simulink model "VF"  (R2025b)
settings: Solver=FixedStepAuto  StartTime=0.0  StopTime=10.0  FixedStep=1e-4  RelTol=1e-3
undefined symbols (not defined in the file): DiscIntNeverNeededParam, Udc
libraries: fl_lib x6, nesl_utility x6, ee_lib x1

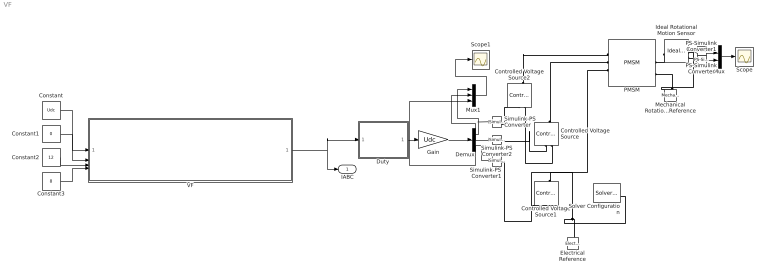
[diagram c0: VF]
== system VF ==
  Constant : Constant  Value=Udc
  Constant1 : Constant  Value=0
  Constant2 : Constant  Value=12
  Constant3 : Constant  Value=8
  Controlled Voltage Source : fl_lib/Electrical/Electrical Sources/Controlled Voltage Source
  Controlled Voltage Source1 : fl_lib/Electrical/Electrical Sources/Controlled Voltage Source
  Controlled Voltage Source2 : fl_lib/Electrical/Electrical Sources/Controlled Voltage Source
  Demux : Demux  Outputs=3
  Duty : Subsystem
  Electrical Reference : fl_lib/Electrical/Electrical Elements/Electrical Reference
  Gain : Gain  Gain=Udc
  Ideal Rotational Motion Sensor : fl_lib/Mechanical/Mechanical Sensors/Ideal Rotational Motion Sensor  reference=foundation.enum.MeasurementReference.difference  acceleration_port=false  velocity_port=true  position_port=true  wrap_angle=false  offset=0 rad
  Mechanical Rotational Reference : fl_lib/Mechanical/Rotational Elements/Mechanical Rotational Reference
  Mux : Mux  Inputs=2
  Mux1 : Mux  Inputs=3
  PMSM : ee_lib/Electromechanical/Permanent Magnet/PMSM  port_option=ee.enum.threePhasePort.expanded  winding_type=ee.enum.electromech.statorconfiguration.wye  machine_param=ee.enum.pmsm.parameterization.constant  nPolePairs=motor.Pn  pmflux_param=ee.enum.pmflux.fluxlinkage  pm_flux_linkage=motor.Flux Wb  torque_constant=0.18 N*m/A  back_emf_constant=0.18 V*s/rad  stator_param=ee.enum.statorparam.LdLqL0  Ld=motor.L H  Lq=motor.L H  idVec=[-200, 0, 200] A  iqVec=[-200, 0, 200] A  LdMatrix=0.0002 * ones(3, 3) H  LqMatrix=0.0002 * ones(3, 3) H  PmMatrix=0.1 * ones(3, 3) Wb  ktMatrix=0.18 * ones(3, 3) N*m/A  keMatrix=0.18 * ones(3, 3) V*s/rad  L0=motor.L H  Ls=0.0002 H  Lm=-0.00002 H  Ms=0.00002 H  Rs=motor.Rs Ohm  zero_sequence=ee.enum.park.zerosequence.include  axes_param=ee.enum.rotorangle.daxis  loss_param=ee.enum.ironloss.none  losses_oc=[0, 0, 0] W  losses_sc=[0, 0, 0] W  f_losses=60 Hz  Isc_losses=95 A  J=75e-6 kg*m^2  lam=8e-5 N*m*s/rad  i_d_specify=off  i_d_priority=None  i_d=0 A  i_d_nominal_specify=off  i_d_nominal_value=1  i_d_nominal_unit=A  i_q_specify=off  i_q_priority=None  i_q=0 A  i_q_nominal_specify=off  i_q_nominal_value=1  i_q_nominal_unit=A  torque_specify=off  torque_priority=None  torque=0 N*m  torque_nominal_specify=off  torque_nominal_value=1  torque_nominal_unit=N*m  angular_velocity_specify=off  angular_velocity_priority=High  angular_velocity=0 rpm  angular_velocity_nominal_specify=off  angular_velocity_nominal_value=1  angular_velocity_nominal_unit=rpm  angular_position_specify=off  angular_position_priority=High  angular_position=0 deg  angular_position_nominal_specify=off  angular_position_nominal_value=1  angular_position_nominal_unit=deg  alpha=3.93e-3 1/K  alpha_flux=-0.001 1/K  Tmeas=298.15 K  stator_thermal_mass=100 J/K  rotor_thermal_mass=200 J/K  Rm_percent_rotor=90  Rd_percent_rotor=30  temperatureA_specify=off  temperatureA_priority=High  temperatureA=25 degC  temperatureA_nominal_specify=off  temperatureA_nominal_value=1  temperatureA_nominal_unit=degC  temperatureB_specify=off  temperatureB_priority=High  temperatureB=25 degC  temperatureB_nominal_specify=off  temperatureB_nominal_value=1  temperatureB_nominal_unit=degC  temperatureC_specify=off  temperatureC_priority=High  temperatureC=25 degC  temperatureC_nominal_specify=off  temperatureC_nominal_value=1  temperatureC_nominal_unit=degC  temperatureR_specify=off  temperatureR_priority=High  temperatureR=25 degC  temperatureR_nominal_specify=off  temperatureR_nominal_value=1  temperatureR_nominal_unit=degC
  PS-Simulink Converter : nesl_utility/PS-Simulink Converter  PhysicalDomain=network_engine_domain  SubClassName=ps_output  LeftPortType=input  RightPortType=output  PseudoPeriodic=off  Frequencies=[]  VectorFormat=inherit  Unit=inherit  AffineConversion=off
  PS-Simulink Converter1 : nesl_utility/PS-Simulink Converter  PhysicalDomain=network_engine_domain  SubClassName=ps_output  LeftPortType=input  RightPortType=output  PseudoPeriodic=off  Frequencies=[]  VectorFormat=inherit  Unit=inherit  AffineConversion=off
  Scope : Scope
  Scope1 : Scope
  Simulink-PS Converter : nesl_utility/Simulink-PS Converter  PhysicalDomain=network_engine_domain  SubClassName=ps_input  LeftPortType=input  RightPortType=output  PseudoPeriodic=off  Frequencies=[]  NoiseDistribution=none  NoiseParameters=[]  Unit=1  AffineConversion=off  FilteringAndDerivatives=provide  SimscapeFilterOrder=1  InputFilterTimeConstant=0.001  UdotUserProvided=0
  Simulink-PS Converter1 : nesl_utility/Simulink-PS Converter  PhysicalDomain=network_engine_domain  SubClassName=ps_input  LeftPortType=input  RightPortType=output  PseudoPeriodic=off  Frequencies=[]  NoiseDistribution=none  NoiseParameters=[]  Unit=1  AffineConversion=off  FilteringAndDerivatives=provide  SimscapeFilterOrder=1  InputFilterTimeConstant=0.001  UdotUserProvided=0
  Simulink-PS Converter2 : nesl_utility/Simulink-PS Converter  PhysicalDomain=network_engine_domain  SubClassName=ps_input  LeftPortType=input  RightPortType=output  PseudoPeriodic=off  Frequencies=[]  NoiseDistribution=none  NoiseParameters=[]  Unit=1  AffineConversion=off  FilteringAndDerivatives=provide  SimscapeFilterOrder=1  InputFilterTimeConstant=0.001  UdotUserProvided=0
  Solver Configuration : nesl_utility/Solver Configuration  PhysicalDomain=network_engine_domain  SubClassName=solver  LeftPortType=input  RightPortType=generic  Tones=[]  Harmonics=[]  SimulateNoise=off  Profile=off  UseLocalSampling=off  EnableSwitchedLinearOptims=on  FrequencyDomain=off  UseCCode=off  RelTol=0.001  AbsTol=0.001  MinStep=1e-09  ToWorkspace=off  RevertToSquareIcSolve=off  NumHomotopyIterations=100  PhasorMode=off  PhasorModeNumHarmonics=1  ConsistencySolver=NEWTON_XTOL_AFTER_FTOL  IndexReductionMethod=DerivativeReplacement  DoDC=off  ResidualTolerance=1e-09  ConsistencyTolSource=GLOBAL  ConsistencyAbsTol=0.001  ConsistencyRelTol=0.001  ConsistencyTolFactor=0.001  UseLocalSolver=off  LocalSolverChoice=NE_BACKWARD_EULER_ADVANCER  ResolveIndetEquations=on  FunctionEvalNumThread=1  LocalSolverSampleTime=0.001  DoFixedCost=off  MaxNonlinIter=3  MaxModeIter=2  ComputeImpulses=off  ImpulseIterations=2  LinearAlgebra=auto  LinearAlgebraNumThread=0  EquationFormulation=NE_TIME_EF  DelaysMemoryBudget=1024  AutomaticFiltering=on  FilteringTimeConstant=0.001  PartitionStorageMethod=AS_NEEDED  PartitionMemoryBudget=1024  PartitionMethod=ROBUST  MultibodyUseLocalSolver=off  MultibodyLocalSolverChoice=ODE1  MultibodyLocalSolverSampleTime=0.001
  VF : Subsystem
  IABC : Outport
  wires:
  Duty/1(DutyOut) -> Gain/1
  Gain/1 -> Demux/1
  Demux/1 -> Mux1/1, Simulink-PS Converter/1
  Demux/2 -> Mux1/2, Simulink-PS Converter2/1
  Demux/3 -> Mux1/3, Simulink-PS Converter1/1
  PS-Simulink Converter/1 -> Mux/1
  PS-Simulink Converter1/1 -> Mux/2
  Mux/1 -> Scope/1
  VF/1(IABC) -> Duty/1(Dutyln), IABC/1
  Constant/1 -> VF/1(v_bus)
  Constant1/1 -> VF/2(ud)
  Constant2/1 -> VF/3(uq)
  Constant3/1 -> VF/4(Freq)
  Mux1/1 -> Scope1/1
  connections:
  Simulink-PS Converter/RConn1 -- Controlled Voltage Source2/RConn1
  Controlled Voltage Source/RConn1 -- Simulink-PS Converter2/RConn1
  Simulink-PS Converter1/RConn1 -- Controlled Voltage Source1/RConn1
  Controlled Voltage Source2/LConn1 -- PMSM/LConn1
  Controlled Voltage Source/LConn1 -- PMSM/LConn2
  Controlled Voltage Source1/LConn1 -- PMSM/LConn3
  Controlled Voltage Source2/RConn2 -- Solver Configuration/RConn1 -- Electrical Reference/LConn1 -- Controlled Voltage Source1/RConn2 -- Controlled Voltage Source/RConn2
  Mechanical Rotational Reference/LConn1 -- Ideal Rotational Motion Sensor/RConn1 -- PMSM/RConn2
  Ideal Rotational Motion Sensor/LConn1 -- PMSM/RConn1
  PS-Simulink Converter1/LConn1 -- Ideal Rotational Motion Sensor/RConn3
  Ideal Rotational Motion Sensor/RConn2 -- PS-Simulink Converter/LConn1

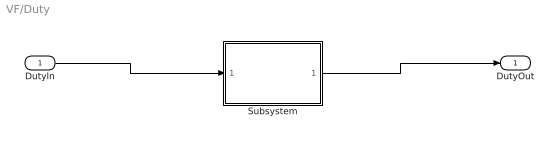
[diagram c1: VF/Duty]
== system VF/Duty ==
  Dutyln : Inport
  Subsystem : Subsystem
  DutyOut : Outport
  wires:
  Dutyln/1 -> Subsystem/1(Dutyln)
  Subsystem/1(DutyOut) -> DutyOut/1

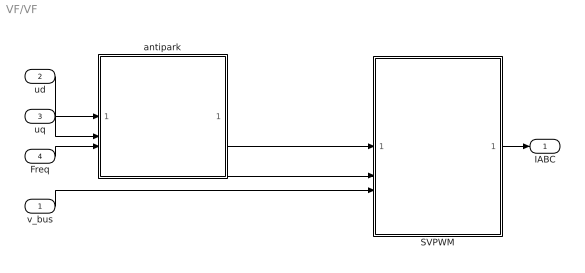
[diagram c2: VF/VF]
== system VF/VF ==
  v_bus : Inport
  ud : Inport  Port=2
  uq : Inport  Port=3
  Freq : Inport  Port=4
  SVPWM : Subsystem
  antipark : Subsystem
  IABC : Outport
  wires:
  v_bus/1 -> SVPWM/3(v_bus)
  ud/1 -> antipark/1(ud)
  antipark/1(ualpha) -> SVPWM/1(Valpha)
  SVPWM/1(IABC) -> IABC/1
  uq/1 -> antipark/2(uq)
  antipark/2(ubeta) -> SVPWM/2(Vbeta)
  Freq/1 -> antipark/3(Freq)

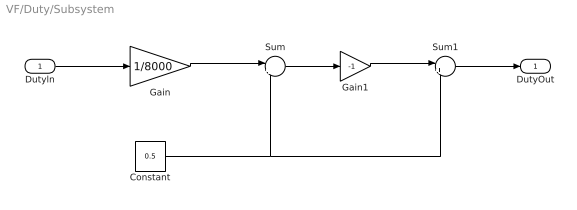
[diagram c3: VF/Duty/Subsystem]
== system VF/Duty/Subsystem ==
  Dutyln : Inport
  Constant : Constant  Value=0.5
  Gain : Gain  Gain=1/8000
  Gain1 : Gain  Gain=-1
  Sum : Sum  Inputs=|+-
  Sum1 : Sum  Inputs=|++
  DutyOut : Outport
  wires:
  Dutyln/1 -> Gain/1
  Constant/1 -> Sum/2, Sum1/2
  Sum1/1 -> DutyOut/1
  Gain/1 -> Sum/1
  Gain1/1 -> Sum1/1
  Sum/1 -> Gain1/1

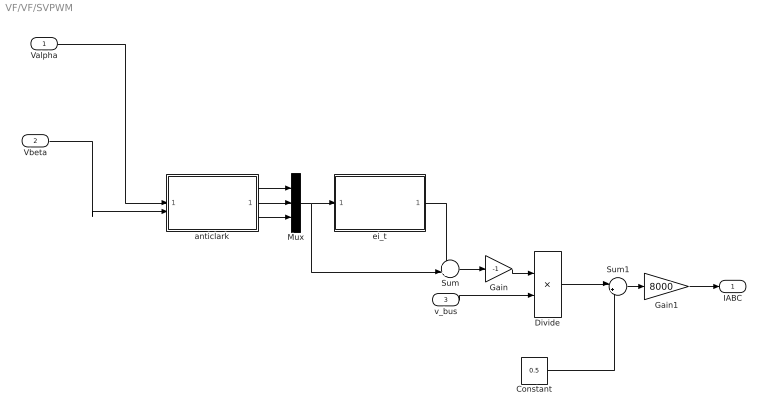
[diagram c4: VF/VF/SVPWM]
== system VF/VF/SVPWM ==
  Valpha : Inport
  Vbeta : Inport  Port=2
  v_bus : Inport  Port=3  OutMin=10
  Constant : Constant  Value=0.5
  Divide : Product  Inputs=*/
  Gain : Gain  Gain=-1
  Gain1 : Gain  Gain=8000
  Mux : Mux  Inputs=3
  Sum : Sum  Inputs=++|
  Sum1 : Sum  Inputs=|++
  anticlark : Subsystem
  ei_t : Subsystem
  IABC : Outport
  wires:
  ei_t/1(ei_t1) -> Sum/1
  Gain1/1 -> IABC/1
  anticlark/2(Vb) -> Mux/2
  Vbeta/1 -> anticlark/2(Vbeta)
  Constant/1 -> Sum1/2
  anticlark/3(Vc) -> Mux/3
  Divide/1 -> Sum1/1
  Sum/1 -> Gain/1
  Gain/1 -> Divide/1
  Sum1/1 -> Gain1/1
  anticlark/1(Va) -> Mux/1
  v_bus/1 -> Divide/2
  Mux/1 -> Sum/2, ei_t/1(Vabc)
  Valpha/1 -> anticlark/1(Valpha)

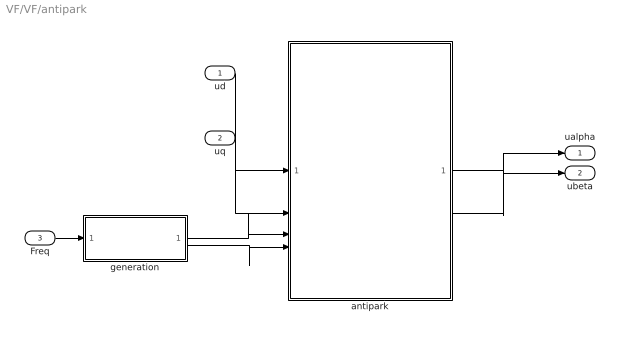
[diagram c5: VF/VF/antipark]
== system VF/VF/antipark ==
  ud : Inport
  uq : Inport  Port=2
  Freq : Inport  Port=3
  antipark : Subsystem
  generation : Subsystem
  ualpha : Outport
  ubeta : Outport  Port=2
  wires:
  generation/2(cos) -> antipark/4(theta_cos)
  generation/1(sin) -> antipark/3(theta_sin)
  antipark/2(ubeta) -> ubeta/1
  antipark/1(ualpha) -> ualpha/1
  ud/1 -> antipark/1(ud)
  uq/1 -> antipark/2(uq)
  Freq/1 -> generation/1(Freq)

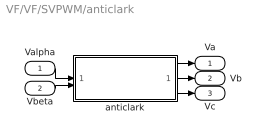
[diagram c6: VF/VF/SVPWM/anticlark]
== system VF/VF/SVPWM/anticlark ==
  Valpha : Inport
  Vbeta : Inport  Port=2
  anticlark : Subsystem
  Va : Outport
  Vb : Outport  Port=2
  Vc : Outport  Port=3
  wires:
  anticlark/3(Vc) -> Vc/1
  Vbeta/1 -> anticlark/2(Vbeta)
  anticlark/1(Va) -> Va/1
  anticlark/2(Vb) -> Vb/1
  Valpha/1 -> anticlark/1(Valpha)

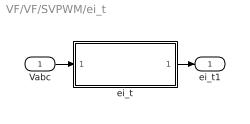
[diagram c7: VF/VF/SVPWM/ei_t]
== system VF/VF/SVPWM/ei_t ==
  Vabc : Inport
  ei_t : Subsystem
  ei_t1 : Outport
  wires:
  Vabc/1 -> ei_t/1(Vabc)
  ei_t/1(ei_t) -> ei_t1/1

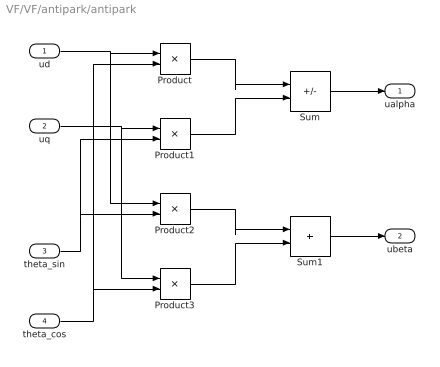
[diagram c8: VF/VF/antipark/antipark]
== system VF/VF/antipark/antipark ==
  ud : Inport
  uq : Inport  Port=2
  theta_sin : Inport  Port=3
  theta_cos : Inport  Port=4
  Product{,1..3} (4 alike) : Product
  Sum : Sum  Inputs=|+-
  Sum1 : Sum  Inputs=|++
  ualpha : Outport
  ubeta : Outport  Port=2
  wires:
  theta_cos/1 -> Product3/2, Product/2
  theta_sin/1 -> Product1/2, Product2/2
  uq/1 -> Product3/1, Product1/1
  ud/1 -> Product2/1, Product/1
  Product/1 -> Sum/1
  Product1/1 -> Sum/2
  Product2/1 -> Sum1/1
  Product3/1 -> Sum1/2
  Sum/1 -> ualpha/1
  Sum1/1 -> ubeta/1

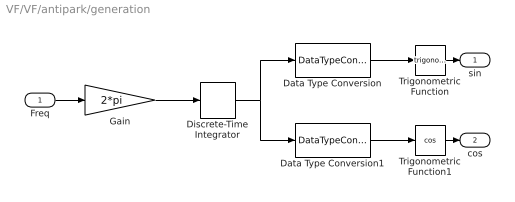
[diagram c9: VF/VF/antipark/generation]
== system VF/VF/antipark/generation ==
  Freq : Inport
  Data Type Conversion : DataTypeConversion  OutDataTypeStr=single
  Data Type Conversion1 : DataTypeConversion  OutDataTypeStr=single
  Discrete-Time Integrator : DiscreteIntegrator  SampleTime=0.0001  ICPrevOutput=DiscIntNeverNeededParam  ICPrevScaledInput=DiscIntNeverNeededParam
  Gain : Gain  Gain=2*pi
  Trigonometric Function : Trigonometry
  Trigonometric Function1 : Trigonometry  Operator=cos
  sin : Outport
  cos : Outport  Port=2
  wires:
  Freq/1 -> Gain/1
  Gain/1 -> Discrete-Time Integrator/1
  Discrete-Time Integrator/1 -> Data Type Conversion1/1, Data Type Conversion/1
  Data Type Conversion/1 -> Trigonometric Function/1
  Data Type Conversion1/1 -> Trigonometric Function1/1
  Trigonometric Function/1 -> sin/1
  Trigonometric Function1/1 -> cos/1

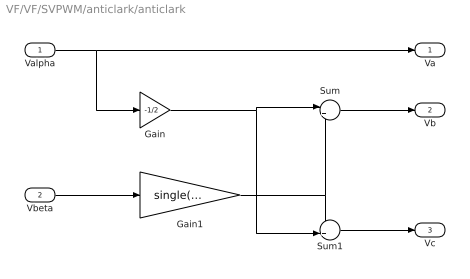
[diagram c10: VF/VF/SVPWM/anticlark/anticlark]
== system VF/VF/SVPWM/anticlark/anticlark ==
  Valpha : Inport
  Vbeta : Inport  Port=2
  Gain : Gain  Gain=-1/2
  Gain1 : Gain  Gain=single(sqrt(3)/2)
  Sum : Sum  Inputs=|++
  Sum1 : Sum  Inputs=-+|
  Va : Outport
  Vb : Outport  Port=2
  Vc : Outport  Port=3
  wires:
  Valpha/1 -> Gain/1, Va/1
  Gain/1 -> Sum1/2, Sum/1
  Gain1/1 -> Sum1/1, Sum/2
  Sum/1 -> Vb/1
  Vbeta/1 -> Gain1/1
  Sum1/1 -> Vc/1

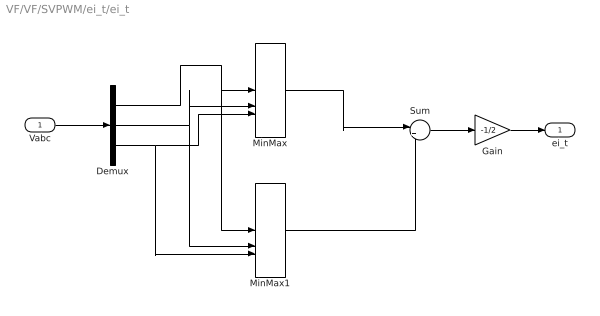
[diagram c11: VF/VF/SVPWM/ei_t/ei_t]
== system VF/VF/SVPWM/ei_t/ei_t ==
  Vabc : Inport
  Demux : Demux  Outputs=3
  Gain : Gain  Gain=-1/2
  MinMax : MinMax  Inputs=3
  MinMax1 : MinMax  Function=max  Inputs=3
  Sum : Sum  Inputs=|++
  ei_t : Outport
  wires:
  Vabc/1 -> Demux/1
  Demux/1 -> MinMax1/1, MinMax/1
  Demux/2 -> MinMax1/2, MinMax/2
  Demux/3 -> MinMax1/3, MinMax/3
  MinMax/1 -> Sum/1
  MinMax1/1 -> Sum/2
  Sum/1 -> Gain/1
  Gain/1 -> ei_t/1
